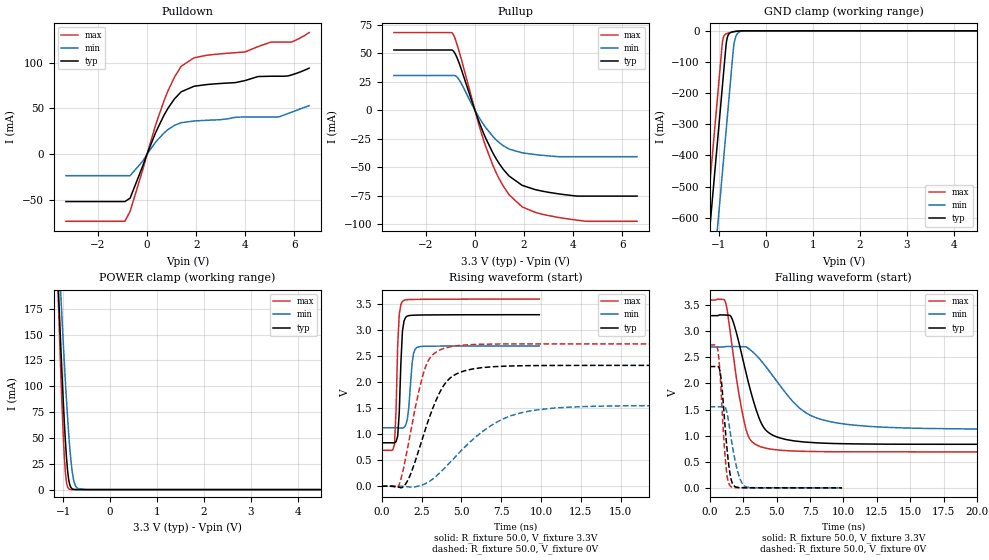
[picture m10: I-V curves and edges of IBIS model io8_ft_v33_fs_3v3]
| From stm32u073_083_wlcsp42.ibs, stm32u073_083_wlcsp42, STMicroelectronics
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[Model]   io8_ft_v33_fs_3v3
Model_type I/O
Polarity   Non-Inverting
Enable   Active-Low
| CAP_THRESHOLD on pad IOFT is "UDTCAPC" :
| Rising=30.0% of vddiom   Falling=70.0% of vddiom
| C_comp min and max val. don't necessarily correlate with the min and max pvt
| but are the smallest and greatest pad capacitance found.
| var   typ   min   max
C_comp   2.27941pF  2.25176pF  2.68142pF
|C_comp_pullup   1.26013pF  1.27540pF  1.50396pF
|C_comp_pulldown   1.01928pF  976.36720fF  1.17746pF
Vinl = 810.0mV
Vinh = 2.52V
Vmeas = 1.65V   | Reference voltage for timing measurements
Cref  = 50.0pF   | Timing specification test load capacitance value
Rref  = 100.0MOhm   | Timing specification test load resistance value
Vref  = 1.65V   | Timing specification test load voltage
[Model Spec]
| TIME_THRESHOLD on pin ZIV33M is "CMOS" :
| Rising=50.0% of vddiom   Falling=50.0% of vddiom
Vinl 1.34770V 1.11470V 1.44970V
Vinh 1.77530V 1.49030V 1.90330V
| variable   typ   min   max
[Temperature Range] 25.0 140.0 -40.0
| variable   typ   min   max
[Voltage Range] 3.3V 2.7V 3.6V
| variable   typ   min   max
[POWER Clamp Reference] 3.3V 2.7V 3.6V
| variable   typ   min   max
[GND Clamp Reference] 0V 0V 0V
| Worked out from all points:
|   slope of the pulldown table from 0 to 0.495 V, typ, clamps not added: 15.6 ohm
|   slope of the pullup table from 0 to 0.495 V, typ, clamps not added: 18.3 ohm
|   GND clamp passes 1 mA (typ) near -0.60 V on its own axis
|   POWER clamp passes 1 mA (typ) near -0.81 V on its own axis
|   rising waveform, R_fixture 50.0, V_fixture 3.3V: 20-80 % time 191ps typ, 251ps min, 182ps max; typ from 0.835 V to 3.3 V
|   falling waveform, R_fixture 50.0, V_fixture 3.3V: 20-80 % time 1.54ns typ, 3.18ns min, 1.06ns max; typ from 3.3 V to 0.835 V
|   rising waveform, R_fixture 50.0, V_fixture 0V: 20-80 % time 1.65ns typ, 3.46ns min, 1.13ns max; typ from 0 V to 2.33 V
|   falling waveform, R_fixture 50.0, V_fixture 0V: 20-80 % time 473ps typ, 665ps min, 395ps max; typ from 2.33 V to 0 V
[POWER Clamp]
-3.3V     2.991A     2.546A     3.694A
-1.11V    202.2mA    242.3mA    190.9mA
-1.09V    180mA      223.6mA    163.4mA
-1.05V    136.9mA    187mA      110.9mA
-1.01V    96.55mA    151.6mA    64.02mA
-970mV    60.39mA    117.9mA    27.41mA
-930mV    31.08mA    86.54mA    7.282mA
-860mV    4.779mA    40.5mA     315.2uA
-810mV    823.2uA    18.15mA    29.21uA
-750mV    88.98uA    4.952mA    1.667uA
-510mV    11.25nA    8.405uA    48.77pA
6.6V      0A         0A         0A
[GND Clamp]
-3.3V     -4.209A    -4.487A    -4.067A
-1.41V    -996.3mA   -1.274A    -854.3mA
-1.25V    -724.3mA   -1.002A    -582.3mA
-1.21V    -656.3mA   -933.6mA   -514.3mA
-930mV    -180.3mA   -457.6mA   -39.53mA
-900mV    -129.3mA   -406.6mA   -18.05mA
-840mV    -33.79mA   -304.6mA   -9.105mA
-790mV    -10.15mA   -219.6mA   -6.665mA
-680mV    -2.476mA   -41.57mA   -2.768mA
-630mV    -1.406mA   -13.77mA   -1.51mA
-530mV    -268.4uA   -1.762mA   -214.9uA
6.6V      830.6pA    196nA      594.5pA
| variable   typ   min   max
[Pullup Reference] 3.3V 2.7V 3.6V
| variable   typ   min   max
[Pulldown Reference] 0V 0V 0V
[Pullup]
-3.3V     52.98mA    30.54mA    68.31mA
-910mV    52.67mA    30.54mA    67.44mA
-810mV    49.8mA     30.45mA    63.04mA
-640mV    41.21mA    26.66mA    51.34mA
200mV     -11.99mA   -7.459mA   -15.6mA
730mV     -37.54mA   -23mA      -48.39mA
980mV     -46.64mA   -28.26mA   -59.98mA
1.39V     -57.81mA   -34.14mA   -74.25mA
1.92V     -65.96mA   -37.41mA   -84.89mA
2.7V      -70.92mA   -39.51mA   -91.15mA
4.29V     -75.45mA   -40.79mA   -96.94mA
6.6V      -75.45mA   -40.79mA   -97.6mA
[Pulldown]
-3.3V     -51.64mA   -23.39mA   -73.18mA
-900mV    -51.64mA   -23.39mA   -73.04mA
-690mV    -47.97mA   -23.39mA   -62.4mA
350mV     23.63mA    13.27mA    31.99mA
690mV     42.49mA    23.17mA    58.21mA
1.12V     60.48mA    31.51mA    84.25mA
1.39V     68.1mA     34.34mA    95.86mA
1.92V     74.17mA    36.28mA    105.3mA
4V        80.41mA    40.64mA    111.6mA
5.39V     85.07mA    40.9mA     122.4mA
5.88V     86.5mA     45.8mA     122.4mA
6.6V      93.9mA     53mA       132.7mA
[Ramp]
dV/dt_r 1.39485V/1.65178ns 931.93627mV/3.45986ns 1.64323V/1.13117ns
dV/dt_f 1.47909V/1.54386ns 946.4517mV/3.1814ns 1.74612V/1.05883ns
R_load = 50.0
| Removed startup time: 0s 0s 0s  .
| Removed end time: 9.9ns.
[Rising Waveform]
R_fixture   = 50.0
V_fixture   = 3.3V
V_fixture_min = 2.7V
V_fixture_max = 3.6V
0s        834.8mV    1.123V     689.8mV
800ps     832.5mV    1.123V     803.3mV
900ps     855.8mV    1.122V     1.467V
1ns       961.1mV    1.122V     2.692V
1.1ns     1.411V     1.121V     3.308V
1.3ns     2.981V     1.119V     3.556V
1.6ns     3.273V     1.275V     3.589V
1.9ns     3.289V     2.345V     3.593V
2.2ns     3.293V     2.668V     3.595V
9.9ns     3.3V       2.7V       3.6V
| Removed startup time: 0s 0s 0s  .
| Removed end time: 49.9ns.
[Falling Waveform]
R_fixture   = 50.0
V_fixture   = 3.3V
V_fixture_min = 2.7V
V_fixture_max = 3.6V
0s        3.3V       2.7V       3.6V
1.1ns     3.312V     2.702V     3.605V
1.6ns     3.283V     2.709V     2.862V
2.2ns     2.773V     2.707V     1.779V
2.8ns     2.119V     2.692V     1.052V
3.6ns     1.404V     2.51V      811.6mV
4.2ns     1.107V     2.325V     760.2mV
7.2ns     876.2mV    1.438V     699mV
10.8ns    842.6mV    1.202V     691mV
49.9ns    834.9mV    1.123V     689.8mV
| Removed startup time: 0s 0s 0s  .
| Removed end time: 49.9ns.
[Rising Waveform]
R_fixture   = 50.0
V_fixture   = 0V
V_fixture_min = 0V
V_fixture_max = 0V
0s        -9.467uV   -14.71uV   3.08uV
1ns       -13.54mV   155uV      -27.52mV
1.5ns     42.71mV    -7.776mV   537.3mV
2.3ns     666.1mV    884.7uV    1.788V
2.8ns     1.151V     57.61mV    2.333V
3.6ns     1.778V     243mV      2.613V
4.3ns     2.082V     461.1mV    2.683V
7.4ns     2.306V     1.261V     2.736V
10.9ns    2.323V     1.504V     2.739V
49.9ns    2.325V     1.553V     2.739V
| Removed startup time: 0s 0s 0s  .
| Removed end time: 9.9ns.
[Falling Waveform]
R_fixture   = 50.0
V_fixture   = 0V
V_fixture_min = 0V
V_fixture_max = 0V
0s        2.325V     1.553V     2.739V
600ps     2.331V     1.553V     2.666V
800ps     2.201V     1.554V     2.106V
1ns       1.686V     1.56V      1.175V
1.2ns     1.023V     1.529V     452.6mV
1.4ns     496.1mV    1.296V     105.6mV
1.6ns     164.4mV    956.6mV    18.42mV
2.1ns     9.02mV     307.6mV    2.787mV
2.7ns     2.704mV    23.06mV    1.593mV
9.9ns     100.2uV    325.3uV    35.46uV
